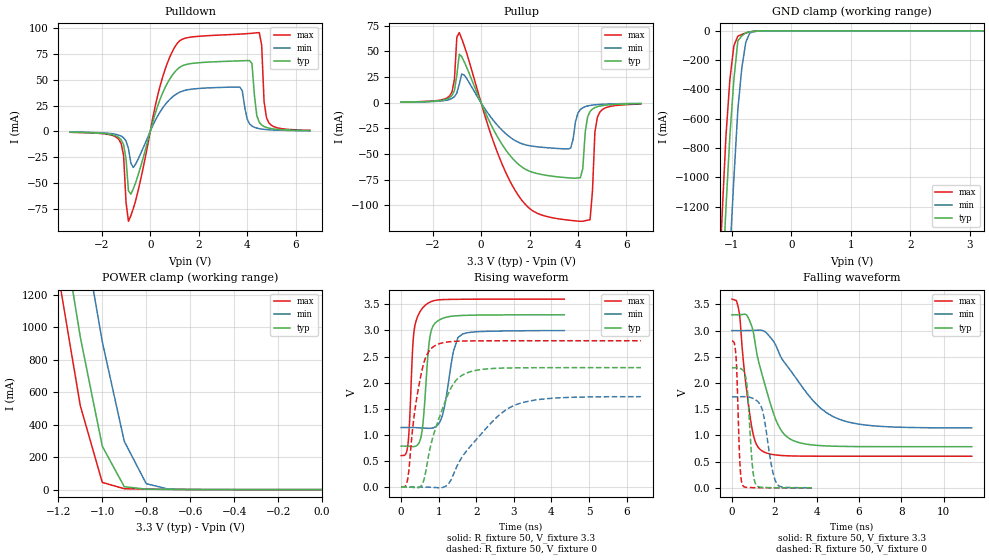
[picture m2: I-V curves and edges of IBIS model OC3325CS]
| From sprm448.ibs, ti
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|   Model Cell OC3325CS
|OC3325CS
[Model]   OC3325CS
Model_type   3-state
Polarity   Non-Inverting
Enable   Active-Low
Cref =  15.0000pF
Rref =  100.0000M
Vref =  0V
Vmeas =  1.65
C_comp   2.5107p   2.136p   3.1702p
[Temperature Range]   25   125   -40
[Voltage Range]   3.3   3   3.6
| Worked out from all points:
|   slope of the pulldown table from 0 to 0.495 V, typ, clamps not added: 13.6 ohm
|   slope of the pullup table from 0 to 0.495 V, typ, clamps not added: 19.6 ohm
|   GND clamp passes 1 mA (typ) near -0.55 V on its own axis
|   POWER clamp passes 1 mA (typ) near -0.67 V on its own axis
|   rising waveform, R_fixture 50, V_fixture 3.3: 20-80 % time 161ps typ, 258ps min, 126ps max; typ from 0.785 V to 3.3 V
|   rising waveform, R_fixture 50, V_fixture 0: 20-80 % time 588ps typ, 1.17ns min, 322ps max; typ from 0 V to 2.29 V
|   falling waveform, R_fixture 50, V_fixture 3.3: 20-80 % time 1ns typ, 2.04ns min, 495ps max; typ from 3.3 V to 0.785 V
|   falling waveform, R_fixture 50, V_fixture 0: 20-80 % time 221ps typ, 413ps min, 139ps max; typ from 2.29 V to 0.001 V
[POWER_clamp]
|   voltage   I(typ)   I(min)   I(max)
-3.3V     22.13A     22.81A     21.76A
-1.2V     1.777A     2.558A     1.326A
-1.167V   1.499A     2.271A     1.056A
-1.133V   1.22A      1.985A     786.7mA
-1.1V     941.2mA    1.698A     517.1mA
-1.067V   716.7mA    1.436A     359.5mA
-1.033V   492.1mA    1.174A     201.9mA
-1V       267.6mA    912.1mA    44.33mA
-900mV    17.82mA    298mA      5.452mA
-800mV    2.597mA    36.49mA    3.097mA
-700mV    1.195mA    3.384mA    1.505mA
-11.55fV  40.21pA    5.882nA    444.1fA
[Pulldown]
|   voltage   I(typ)   I(min)   I(max)
-3.3V     -841.7uA   -670.2uA   -911.7uA
-1.3V     -5.851mA   -3.631mA   -7.716mA
-1.1V     -12.99mA   -6.25mA    -23.49mA
-900mV    -57.69mA   -16.71mA   -87.36mA
-700mV    -55.83mA   -35.1mA    -75.12mA
1.1V      59.92mA    36.57mA    85.06mA
3.7V      68.51mA    42.93mA    94.48mA
4.1V      68.8mA     7.362mA    95.13mA
4.5V      8.911mA    2.645mA    95.99mA
4.7V      4.671mA    1.979mA    28.88mA
4.9V      3.124mA    1.577mA    8.243mA
6.6V      798.5uA    571.1uA    1.034mA
[Pullup]
|   voltage   I(typ)   I(min)   I(max)
-3.3V     669.2uA    562.7uA    746.5uA
-1.3V     4.957mA    3.263mA    6.677mA
-1.1V     12mA       5.961mA    22.79mA
-1V       26.99mA    9.54mA     64.01mA
-900mV    47.32mA    18.06mA    68.43mA
1.5V      -59.02mA   -37.99mA   -88.89mA
3.7V      -73.26mA   -44.09mA   -114.6mA
4.1V      -72.89mA   -6.562mA   -115.5mA
4.5V      -8.453mA   -2.591mA   -113.8mA
4.7V      -4.667mA   -1.97mA    -28.55mA
4.9V      -3.189mA   -1.585mA   -9.195mA
6.6V      -843.6uA   -589.3uA   -1.225mA
[GND_clamp]
|   voltage   I(typ)   I(min)   I(max)
-3.3V     -22.45A    -23.24A    -22.02A
-1.233V   -2.371A    -3.249A    -1.858A
-1.167V   -1.782A    -2.654A    -1.277A
-1.1V     -1.21A     -2.069A    -719.9mA
-1.033V   -714.3mA   -1.52A     -330.2mA
-966.7mV  -333.9mA   -1.01A     -102.4mA
-900mV    -68.71mA   -538.7mA   -36.21mA
-833.3mV  -34.32mA   -253.8mA   -24.9mA
-766.7mV  -13.76mA   -79.03mA   -15.2mA
-700mV    -7.006mA   -14.27mA   -7.097mA
-433.3mV  -71.75uA   -256uA     -23.2uA
3.233V    37.53pA    1.424uA    386.4fA
[Ramp]
| variable   typ   min   max
dV/dt_f   1.516009/1.004885n   1.120176/2.044922n   1.808099/0.4951693n
dV/dt_r   1.381596/0.5892205n   1.048423/1.172127n   1.690797/0.3215311n
R_load = 50
[Rising Waveform]
R_fixture = 50
V_fixture = 3.3
V_fixture_min = 3
V_fixture_max = 3.6
|   time   V(typ)   V(min)   V(max)
0s        785.3mV    1.141V     603.3mV
184ps     782.2mV    1.142V     835.3mV
360ps     778.7mV    1.14V      3.071V
520ps     933.5mV    1.135V     3.379V
624ps     1.591V     1.13V      3.47V
776ps     2.919V     1.126V     3.545V
1ns       3.194V     1.215V     3.586V
1.392ns   3.276V     2.602V     3.596V
1.64ns    3.287V     2.934V     3.597V
4.344ns   3.299V     2.997V     3.6V
[Rising Waveform]
R_fixture = 50
V_fixture = 0
V_fixture_min = 0
V_fixture_max = 0
|   time   V(typ)   V(min)   V(max)
0s        46.36pV    15.58nV    1.512pV
176ps     600.4uV    127.7uV    159.9mV
344ps     -7.556mV   295.5uV    1.354V
544ps     36.26mV    448.2uV    2.202V
904ps     1.099V     -7.493mV   2.71V
1.408ns   1.996V     269.4mV    2.79V
1.872ns   2.216V     804.6mV    2.8V
2.608ns   2.277V     1.379V     2.802V
3.232ns   2.285V     1.619V     2.803V
6.384ns   2.288V     1.732V     2.803V
[Falling Waveform]
R_fixture = 50
V_fixture = 3.3
V_fixture_min = 3
V_fixture_max = 3.6
|   time   V(typ)   V(min)   V(max)
0s        3.3V       3V         3.6V
352ps     3.303V     3V         3.323V
760ps     3.254V     3.001V     1.645V
1.08ns    2.8V       3.005V     907.3mV
1.432ns   2.149V     3.003V     702.7mV
2.176ns   1.204V     2.621V     622.8mV
3.032ns   881.1mV    2.09V      607.2mV
4.2ns     805.5mV    1.517V     603.7mV
5.392ns   790mV      1.266V     603.3mV
11.34ns   785.4mV    1.144V     603.3mV
[Falling Waveform]
R_fixture = 50
V_fixture = 0
V_fixture_min = 0
V_fixture_max = 0
|   time   V(typ)   V(min)   V(max)
0s        2.289V     1.735V     2.803V
192ps     2.293V     1.736V     2.498V
384ps     2.28V      1.739V     397.1mV
496ps     2.253V     1.74V      56.14mV
704ps     1.968V     1.737V     8.864mV
944ps     513.4mV    1.714V     4.92mV
1.136ns   57.14mV    1.673V     3.459mV
1.464ns   8.864mV    1.44V      2.144mV
2.128ns   2.964mV    74.35mV    837.4uV
3.776ns   763.7uV    3.017mV    145.8uV
